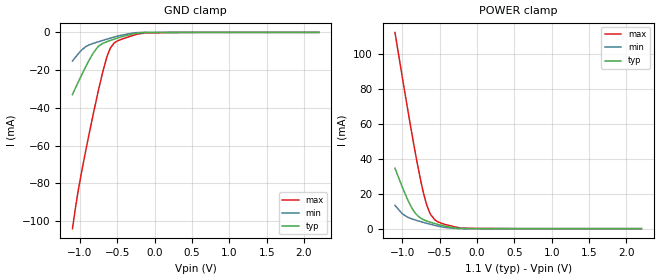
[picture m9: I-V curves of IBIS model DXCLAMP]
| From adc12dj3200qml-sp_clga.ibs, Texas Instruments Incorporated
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[Model]   DXCLAMP
Model_type   Terminator
|   typ   min   max
C_comp   2.87pF   2.8pF   2.93pF
[Voltage Range]   1.1   1.05   1.15
[Temperature Range]   25   125   -40
[Pullup Reference]   1.1   1.05   1.15
[Pulldown Reference]   0   0   0
[Power Clamp Reference]   1.1   1.05   1.15
[GND Clamp Reference]   0   0   0
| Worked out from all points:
|   GND clamp passes 1 mA (typ) near -0.31 V on its own axis
|   POWER clamp passes 1 mA (typ) near -0.38 V on its own axis
[GND Clamp]
|   Voltage   I(typ)   I(min)   I(max)
-1.1V     -32.91mA   -15.17mA   -104mA
-1.024V   -26.4mA    -11.4mA    -84.07mA
-977.9mV  -22.59mA   -9.393mA   -73.93mA
-826.1mV  -11.21mA   -5.882mA   -44.07mA
-750.2mV  -7.306mA   -4.923mA   -30.24mA
-690.8mV  -5.757mA   -4.198mA   -20.34mA
-631.4mV  -4.813mA   -3.488mA   -12.09mA
-591.8mV  -4.257mA   -3.027mA   -8.234mA
-539mV    -3.545mA   -2.431mA   -5.531mA
-275mV    -634.6uA   -246.7uA   -1.388mA
-103.4mV  -61.29uA   -10.1uA    -306.9uA
2.2V      0A         0A         0A
[POWER Clamp]
|   Voltage   I(typ)   I(min)   I(max)
-1.1V     34.61mA    13.36mA    112.5mA
-1.004V   24.09mA    8.661mA    87.39mA
-888.8mV  13.03mA    5.832mA    58.12mA
-826.1mV  8.805mA    4.935mA    43.08mA
-743.6mV  5.707mA    3.883mA    25.17mA
-710.6mV  5.001mA    3.481mA    19.09mA
-671mV    4.346mA    3.011mA    13.12mA
-621.5mV  3.643mA    2.45mA     8.023mA
-562.1mV  2.866mA    1.82mA     4.87mA
-430.1mV  1.367mA    683.2uA    2.428mA
-159.5mV  59.95uA    11.57uA    271.3uA
2.2V      0A         0A         0A
